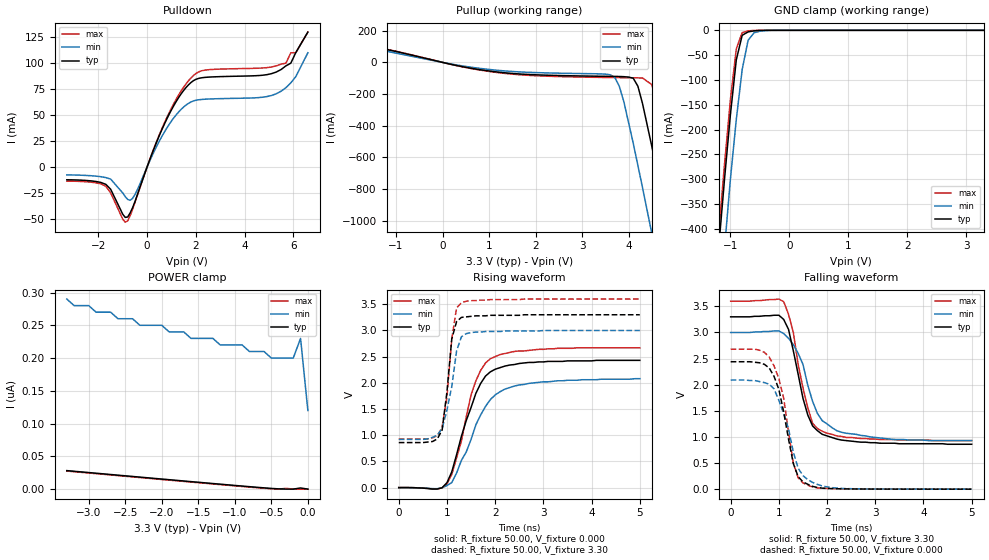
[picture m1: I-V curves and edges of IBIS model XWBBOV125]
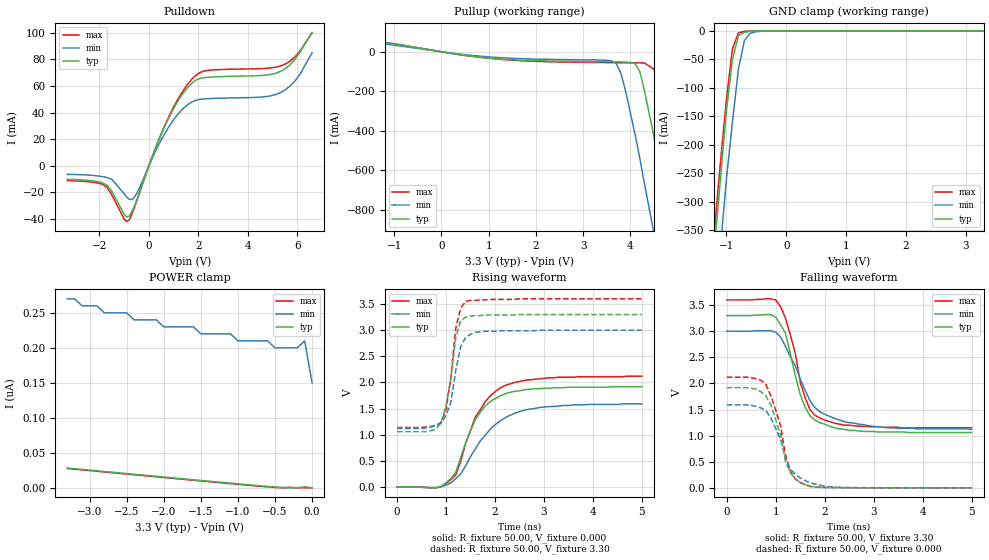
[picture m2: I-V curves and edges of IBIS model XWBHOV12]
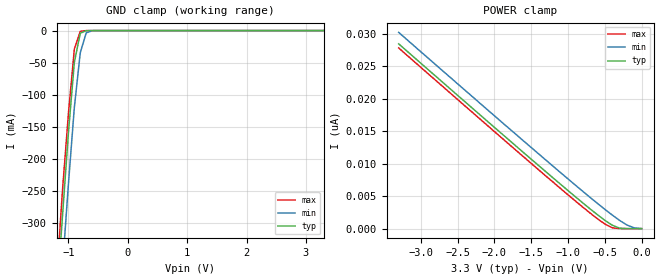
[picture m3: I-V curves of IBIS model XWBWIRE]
|   National Semiconductor Corporation
|   Networks Division
|   IBIS Model for DP83846A
|   80 Pin LQFP Package
| IBIS file dp83846a.ibs was created using s2ibis2 version 2.1
| North Carolina State University Electronics Research Laboratory 1997
| http://www.eigroup.org/ibis/tools.htm -> SPICE-toIBISconversion(IBISv2.1)
| s2ibis2.tar.Z   11FEB97   652K
| s2ibis2_fix.tar.Z 13MAY97   119K
[IBIS ver]   2.1
[File name]   dp83846a.ibs
[File Rev]   2.0
[Date]   17APR01
[Source]   National Semiconductor Corporation, Networks Division
[Notes]   For questions or comments contact
   Alan.E.Segervall@nsc.com or phone 408-721-7082
   Spectre s2ibis simulations, created by Alan E Segervall.
| Due to IBIS modeling limitations and design complexity this model
| does not support the Ethernet Transmit Data pins:
| [Pin]   signal_name   model_name
| 16  TD+   NC   0.321   4.888nH   0.078pF
| 17  TD-   NC   0.336   5.093nH   0.082pF
| Please refer to product datasheet and application notes for PC board
| layout recommendations.
[Disclaimer]  Absolutely no guarantees, for modeling purposes only.
   National Semiconductor Corporation hereby grants the user of this IBIS
model a non-exclusive, nontransferable license to use this IBIS model under
the following terms. Before using this IBIS model, the user should read this
license.  If the user does not accept these terms,  the IBIS model should be
returned to National within 30 days.
   The user is granted this license only to use the IBIS model and is not
granted rights to sell, load, rent, lease or license the IBIS model in whole
or in part, or in modified form to anyone other than user. User may modify
the IBIS model to suit its specific applications but rights to derivative
works and such modifications shall belong to National.
   This IBIS model is provided on an "AS IS" basis and National makes
absolutely no warranty with respect to the information contained herein.
NATIONAL DISCLAIMS AND CUSTOMER WAIVES ALL WARRANTIES, EXPRESS OR IMPLIED,
INCLUDING WARRANTIES OF MERCHANTABILITY OR FITNESS FOR A PARTICULAR PURPOSE.
The entire risk as to quality and performance is with the Customer.
ACCORDINGLY, IN NO EVENT SHALL THE COMPANY BE LIABLE FOR ANY DAMAGES, WHETHER
IN CONTRACT OR COURT, INCLUDING ANY LOST PROFITS OR OTHER INCIDENTAL,
CONSEQUENTIAL, EXEMPLARY, OR PUNITIVE DAMAGES ARISING OUT OF THE USE OR
APPLICATION OF THE IBIS model provided in this package. Further, National
reserves the right to make changes without notice to any product herein to
improve reliability, function, or design. National does not convey any license
under patent rights or any other intellectual property rights, including those
of third parties.
   National is not obligated to provide maintenance or support
for the licensed IBIS model.
[Copyright]   Copyright 2001, National Semiconductor Corporation, All rights
   reserved
|   Component DP83846A
[Component]   DP83846A
[Manufacturer]   National Semiconductor Corporation
[Package]
| variable   typ   min   max
R_pkg   0.333   0.287   0.382
L_pkg   5.049nH   4.529nH   5.845nH
C_pkg   0.106pF   0.078pF   0.283pF
[Pin] signal_name   model_name   R_pin   L_pin   C_pin
1   RESERVED   NC   0.382   5.845nH   0.283pF
2   ANA_GND1   GND   0.375   5.634nH   0.109pF
3   RBIAS   XWBWIRE   0.362   5.447nH   0.089pF
4   ANA_VDD1   POWER   0.350   5.273nH   0.082pF
5   RESERVED   NC   0.340   5.129nH   0.080pF
6   ANA_GND2   GND   0.332   4.986nH   0.078pF
7   ANA_VDD2   POWER   0.326   4.877nH   0.078pF
8   RESERVED   XWBWIRE   0.320   4.796nH   0.082pF
9   ANA_GND3   GND   0.314   4.751nH   0.091pF
10  RD-   RD   0.304   4.746nH   0.091pF
11  RD+   RD   0.287   4.529nH   0.090pF
12  ANA_VDD3   POWER   0.297   4.540nH   0.089pF
13  ANA_GND4   GND   0.303   4.576nH   0.080pF
14  ANA_VDD4   POWER   0.306   4.650nH   0.079pF
15  ANA_GND5   GND   0.313   4.753nH   0.078pF
16  TD+   NC   0.321   4.888nH   0.078pF
17  TD-   NC   0.336   5.093nH   0.082pF
18  ANA_GND6   GND   0.350   5.279nH   0.089pF
19  SUB_GND1   GND   0.363   5.480nH   0.106pF
20  RESERVED   NC   0.371   5.716nH   0.281pF
21  RESERVED   XWBBOV125   0.382   5.845nH   0.283pF
22  RESERVED   XWBBOV125   0.375   5.634nH   0.109pF
23  CORE_GND1   GND   0.362   5.447nH   0.089pF
24  CORE_VDD1   POWER   0.350   5.273nH   0.082pF
25  AN_0   XWBBOV125   0.340   5.129nH   0.080pF
26  AN_1   XWBBOV125   0.332   4.986nH   0.078pF
27  AN_EN   XWBBOV62   0.326   4.877nH   0.078pF
28  LED_SPEED   XWBBOV62   0.320   4.796nH   0.082pF
29  LED_RX/PADDR4   XWBBOV62   0.314   4.751nH   0.091pF
30  LED_TX/PADDR3   XWBBOV62   0.304   4.746nH   0.091pF
31  LED_GDLNK/PADDR2   XWBBOV125   0.287   4.529nH   0.090pF
32  LED_COL/PADDR1   XWBBOV62   0.297   4.540nH   0.089pF
33  LED_FDPLX/PADDR0   XWBBOV62   0.303   4.576nH   0.080pF
34  IO_GND   GND   0.306   4.650nH   0.079pF
35  IO_VDD   POWER   0.313   4.753nH   0.078pF
36  MDIO   XWBHOV12   0.321   4.888nH   0.078pF
37  MDC   XWBHOV12   0.336   5.093nH   0.082pF
38  RXD_3/CD_RF1   XWBBOV62   0.350   5.279nH   0.089pF
39  RXD_2/CD_RF0   XWBBOV62   0.363   5.480nH   0.106pF
40  RXD_1/CRM_LF_SEL   XWBBOV125   0.371   5.716nH   0.281pF
41  RXD_0/FCO_EN   XWBBOV125   0.382   5.845nH   0.283pF
42  IO_GND   GND   0.375   5.634nH   0.109pF
43  IO_VDD   POWER   0.362   5.447nH   0.089pF
44  RX_DV   XWBBOV62   0.350   5.273nH   0.082pF
45  RX_CLK   XWBBOV62   0.340   5.129nH   0.080pF
46  RX_ER/PAUSE_EN   XWBBOV62   0.332   4.986nH   0.078pF
47  RESERVED   XWBBOV125   0.326   4.877nH   0.078pF
48  CORE_GND2   GND   0.320   4.796nH   0.082pF
49  CORE_VDD2   POWER   0.314   4.751nH   0.091pF
50  TX_ER   XWBHOV12   0.304   4.746nH   0.091pF
51  TX_CLK   XWBHOV12   0.287   4.529nH   0.090pF
52  TX_EN   XWBHOV12   0.297   4.540nH   0.089pF
53  IO_GND3   GND   0.303   4.576nH   0.080pF
54  TXD_0   XWBHOV12   0.306   4.650nH   0.079pF
55  TXD_1   XWBHOV12   0.313   4.753nH   0.078pF
56  IO_GND4   GND   0.321   4.888nH   0.078pF
57  IO_VDD4   POWER   0.336   5.093nH   0.082pF
58  TXD_2   XWBHOV12   0.350   5.279nH   0.089pF
59  TXD_3   XWBHOV12   0.363   5.480nH   0.106pF
60  COL   XWBHOV12   0.371   5.716nH   0.281pF
61  CRS/LED_CFG   XWBHOV12   0.382   5.845nH   0.283pF
62  RESET   XWBHOV12   0.375   5.634nH   0.109pF
63  RESERVED   XWBHOV12   0.362   5.447nH   0.089pF
64  IO_GND5   GND   0.350   5.273nH   0.082pF
65  IO_VDD5   POWER   0.340   5.129nH   0.080pF
66  X2   OSC25_XO   0.332   4.986nH   0.078pF
67  X1   OSC25_XI   0.326   4.877nH   0.078pF
68  RESERVED   XWBHOV12   0.320   4.796nH   0.082pF
69  RESERVED   XWBHOV12   0.314   4.751nH   0.091pF
70  RESERVED   XWBHOV12   0.304   4.746nH   0.091pF
71  RESERVED   XWBHOV12   0.287   4.529nH   0.090pF
72  CORE_VDD3   POWER   0.297   4.540nH   0.089pF
73  CORE_GND3   GND   0.303   4.576nH   0.080pF
74  RESERVED   NC   0.306   4.650nH   0.079pF
75  RESERVED   NC   0.313   4.753nH   0.078pF
76  SUB_GND2   GND   0.321   4.888nH   0.078pF
77  RESERVED   NC   0.336   5.093nH   0.082pF
78  RESERVED   NC   0.350   5.279nH   0.089pF
79  SUB_GND3   GND   0.363   5.480nH   0.106pF
80  RESERVED   NC   0.371   5.716nH   0.281pF
[Diff Pin]  inv_pin  vdiff   tdelay_typ
11   10   0.100V   0.000s
16   17   0.000V   0.000s
| Models and submodels in the file (7): XWBBOV125 (I/O), XWBHOV12 (I/O), XWBWIRE (Input), RD (Input), XWBBOV62 (I/O), OSC25_XO (Output), OSC25_XI (Input)
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|   Model XWBBOV125
[Model]   XWBBOV125
Model_type   I/O
Polarity   Non-Inverting
Enable   Active-High
Vinl =   0.80V
Vinh =   2.00V
Vmeas =   1.50V
Cref =  20.00pF
Rref = 100.00k
C_comp   5.00pF   5.00pF   5.00pF
[Temperature Range]   25.00   0.14k   0.000
[Voltage Range]   3.30V   3.00V   3.60V
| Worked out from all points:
|   slope of the pulldown table from 0 to 0.495 V, typ, clamps not added: 16.5 ohm
|   slope of the pullup table from 0 to 0.495 V, typ, clamps not added: 16.1 ohm
|   GND clamp passes 1 mA (typ) near -0.58 V on its own axis
|   rising waveform, R_fixture 50.00, V_fixture 0.000: 20-80 % time 519ps typ, 631ps min, 459ps max; typ from 0 V to 2.43 V
|   rising waveform, R_fixture 50.00, V_fixture 3.30: 20-80 % time 163ps typ, 237ps min, 185ps max; typ from 0.86 V to 3.3 V
|   falling waveform, R_fixture 50.00, V_fixture 3.30: 20-80 % time 374ps typ, 469ps min, 351ps max; typ from 3.3 V to 0.86 V
|   falling waveform, R_fixture 50.00, V_fixture 0.000: 20-80 % time 318ps typ, 383ps min, 304ps max; typ from 2.44 V to 0 V
[Pulldown]
| voltage   I(typ)   I(min)   I(max)
-3.3V     -12.55mA   -7.84mA    -13.87mA
-1.7V     -16.93mA   -10.43mA   -18.73mA
-1V       -45.94mA   -25.36mA   -50.67mA
-800mV    -48.46mA   -31.53mA   -52.2mA
-500mV    -33.54mA   -26.73mA   -34.28mA
700mV     40.82mA    33.24mA    41.89mA
1.8V      81.34mA    62.58mA    85.74mA
5.3V      91.41mA    70.44mA    97.34mA
5.7V      97.44mA    76.39mA    100mA
5.9V      100mA      81mA       110mA
6.1V      110mA      86.86mA    110mA
6.6V      130mA      110mA      130mA
[Pullup]
| voltage   I(typ)   I(min)   I(max)
-3.3V     200mA      170mA      210mA
900mV     -50.23mA   -41.2mA    -52.73mA
3.6V      -88.17mA   -77.79mA   -95.51mA
3.8V      -89.02mA   -150mA     -96.22mA
3.9V      -90.24mA   -250mA     -96.54mA
4.1V      -99.71mA   -510mA     -97.17mA
4.3V      -260mA     -790mA     -98.85mA
4.5V      -530mA     -1.08A     -140mA
4.9V      -1.12A     -1.67A     -650mA
5.1V      -1.42A     -1.97A     -950mA
5.3V      -1.73A     -2.28A     -1.25A
6.6V      -3.73A     -4.26A     -3.25A
[GND_clamp]
| voltage   I(typ)   I(min)   I(max)
-3.3V     -3.64A     -3.72A     -3.62A
-1.2V     -440mA     -570mA     -410mA
-1.1V     -300mA     -440mA     -270mA
-1V       -170mA     -300mA     -140mA
-900mV    -59.59mA   -180mA     -37.47mA
-800mV    -10.05mA   -78.91mA   -4.5mA
-700mV    -3.19mA    -20.3mA    -1.15mA
-600mV    -1.14mA    -5.01mA    -210uA
-500mV    -210uA     -1.78mA    -18.22uA
-200mV    -44.3nA    -11.19uA   -980pA
3.3V      93.97pA    200nA      36.14pA
[POWER_clamp]
| voltage   I(typ)   I(min)   I(max)
-3.3V     28.33nA    290nA      27.68nA
-2.7V     22.38nA    270nA      21.73nA
-2.6V     21.39nA    260nA      20.74nA
-2.4V     19.41nA    260nA      18.76nA
-2.3V     18.42nA    250nA      17.77nA
-2V       15.46nA    250nA      14.81nA
-1.6V     11.54nA    230nA      10.88nA
-900mV    4.78nA     220nA      4.12nA
-500mV    1.18nA     200nA      630pA
-200mV    120pA      200nA      190pA
-100mV    1.86nA     230nA      45.35pA
0V        93.97pA    120nA      39.6pA
[Ramp]
| variable   typ   min   max
dV/dt_r   1.92/0.26n   1.74/0.34n   2.10/0.26n
dV/dt_f   1.92/0.27n   1.73/0.37n   2.10/0.26n
R_load = 0.50k
[Rising Waveform]
R_fixture = 50.00
V_fixture = 0.000
V_fixture_min = 0.000
V_fixture_max = 0.000
| time   V(typ)   V(min)   V(max)
0s        130uV      110uV      140uV
800ps     -25.56mV   -20.49mV   -29.57mV
1ns       93.95mV    39.4mV     72.64mV
1.1ns     300mV      96.74mV    250mV
1.3ns     980mV      520mV      890mV
1.5ns     1.53V      920mV      1.77V
1.6ns     1.8V       1.2V       2.04V
1.9ns     2.21V      1.68V      2.46V
2.7ns     2.39V      1.99V      2.62V
5ns       2.43V      2.08V      2.67V
[Rising Waveform]
R_fixture = 50.00
V_fixture = 3.30
V_fixture_min = 3.00
V_fixture_max = 3.60
| time   V(typ)   V(min)   V(max)
0s        860mV      920mV      930mV
700ps     880mV      960mV      950mV
800ps     930mV      1V         990mV
900ps     1.1V       1.13V      1.15V
1ns       1.83V      1.48V      1.74V
1.1ns     2.84V      1.93V      2.84V
1.2ns     3.17V      2.61V      3.43V
1.3ns     3.25V      2.88V      3.53V
1.8ns     3.28V      2.98V      3.58V
5ns       3.3V       3V         3.6V
[Falling Waveform]
R_fixture = 50.00
V_fixture = 3.30
V_fixture_min = 3.00
V_fixture_max = 3.60
| time   V(typ)   V(min)   V(max)
0s        3.3V       3V         3.6V
1.1ns     3.25V      2.98V      3.59V
1.2ns     3.06V      2.89V      3.35V
1.3ns     2.65V      2.77V      3V
1.5ns     1.74V      2.39V      1.94V
1.6ns     1.42V      1.99V      1.56V
1.7ns     1.21V      1.68V      1.26V
1.8ns     1.12V      1.45V      1.16V
2.4ns     930mV      1.07V      990mV
5ns       860mV      930mV      930mV
[Falling Waveform]
R_fixture = 50.00
V_fixture = 0.000
V_fixture_min = 0.000
V_fixture_max = 0.000
| time   V(typ)   V(min)   V(max)
0s        2.44V      2.09V      2.68V
600ps     2.42V      2.06V      2.66V
900ps     2.16V      1.92V      2.36V
1ns       1.91V      1.7V       2.12V
1.1ns     1.48V      1.45V      1.74V
1.3ns     490mV      710mV      500mV
1.4ns     240mV      400mV      220mV
1.5ns     140mV      260mV      120mV
2.2ns     8.79mV     21.51mV    9.2mV
5ns       240uV      370uV      270uV
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|   Model XWBHOV12
[Model]   XWBHOV12
Model_type   I/O
Polarity   Non-Inverting
Enable   Active-High
Vinl =   0.80V
Vinh =   2.00V
Vmeas =   1.50V
Cref =  20.00pF
Rref = 100.00k
C_comp   5.00pF   5.00pF   5.00pF
[Temperature Range]   25.00   0.14k   0.000
[Voltage Range]   3.30V   3.00V   3.60V
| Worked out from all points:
|   slope of the pulldown table from 0 to 0.495 V, typ, clamps not added: 21.1 ohm
|   slope of the pullup table from 0 to 0.495 V, typ, clamps not added: 28 ohm
|   GND clamp passes 1 mA (typ) near -0.60 V on its own axis
|   rising waveform, R_fixture 50.00, V_fixture 0.000: 20-80 % time 551ps typ, 775ps min, 585ps max; typ from 0 V to 1.92 V
|   rising waveform, R_fixture 50.00, V_fixture 3.30: 20-80 % time 212ps typ, 237ps min, 193ps max; typ from 1.06 V to 3.3 V
|   falling waveform, R_fixture 50.00, V_fixture 3.30: 20-80 % time 397ps typ, 612ps min, 395ps max; typ from 3.3 V to 1.06 V
|   falling waveform, R_fixture 50.00, V_fixture 0.000: 20-80 % time 336ps typ, 408ps min, 340ps max; typ from 1.92 V to 0 V
[Pulldown]
| voltage   I(typ)   I(min)   I(max)
-3.3V     -10.21mA   -6.41mA    -11.24mA
-1.7V     -14.38mA   -8.76mA    -15.95mA
-900mV    -38.4mA    -23.38mA   -41.84mA
-700mV    -34.77mA   -25.38mA   -36.84mA
-500mV    -26.29mA   -20.89mA   -26.78mA
800mV     35.83mA    29.09mA    36.68mA
1.3V      52.23mA    41.38mA    54.01mA
1.8V      62.95mA    48.5mA     66.19mA
2.4V      66.48mA    50.41mA    71.64mA
5.3V      70.67mA    54.75mA    74.83mA
5.9V      79.7mA     63.54mA    81.56mA
6.6V      100mA      84.8mA     100mA
[Pullup]
| voltage   I(typ)   I(min)   I(max)
-3.3V     110mA      27.65mA    110mA
-2.7V     96.2mA     77.73mA    99.58mA
1V        -31.19mA   -25.59mA   -32.8mA
3.6V      -50.7mA    -46.05mA   -54.92mA
3.8V      -51.25mA   -110mA     -55.32mA
4.1V      -59.9mA    -420mA     -55.87mA
4.3V      -200mA     -670mA     -57.12mA
4.5V      -430mA     -920mA     -88.04mA
4.9V      -950mA     -1.44A     -540mA
5.1V      -1.21A     -1.7A      -800mA
5.3V      -1.48A     -1.97A     -1.06A
6.6V      -3.23A     -3.7A      -2.81A
[GND_clamp]
| voltage   I(typ)   I(min)   I(max)
-3.3V     -3.18A     -3.26A     -3.16A
-1.2V     -380mA     -500mA     -350mA
-1.1V     -260mA     -380mA     -230mA
-1V       -140mA     -260mA     -120mA
-900mV    -50.62mA   -160mA     -31.57mA
-800mV    -8.35mA    -67.12mA   -3.69mA
-700mV    -2.68mA    -16.92mA   -950uA
-600mV    -980uA     -4.21mA    -170uA
-500mV    -190uA     -1.55mA    -15.48uA
-200mV    -43.2nA    -10.78uA   -890pA
3.3V      110pA      200nA      36.28pA
[POWER_clamp]
| voltage   I(typ)   I(min)   I(max)
-3.3V     28.34nA    270nA      27.68nA
-2.8V     23.38nA    250nA      22.72nA
-2V       15.48nA    230nA      14.81nA
-1.6V     11.55nA    230nA      10.88nA
-1.5V     10.58nA    220nA      9.91nA
-1.1V     6.7nA      220nA      6.03nA
-1V       5.74nA     210nA      5.07nA
-600mV    2.04nA     210nA      1.4nA
-500mV    1.2nA      200nA      630pA
-200mV    130pA      200nA      130pA
-100mV    1.59nA     210nA      43.62pA
0V        110pA      150nA      39.7pA
[Ramp]
| variable   typ   min   max
dV/dt_r   1.88/0.28n   1.69/0.38n   2.06/0.28n
dV/dt_f   1.90/0.29n   1.72/0.41n   2.08/0.28n
R_load = 0.50k
[Rising Waveform]
R_fixture = 50.00
V_fixture = 0.000
V_fixture_min = 0.000
V_fixture_max = 0.000
| time   V(typ)   V(min)   V(max)
0s        89.13uV    78.2uV     98.24uV
800ps     -12.15mV   -8.36mV    -14.42mV
1.1ns     160mV      77.86mV    140mV
1.2ns     280mV      160mV      230mV
1.4ns     840mV      400mV      830mV
1.6ns     1.29V      730mV      1.34V
1.9ns     1.63V      1.1V       1.74V
2.2ns     1.78V      1.32V      1.94V
3.1ns     1.89V      1.54V      2.09V
5ns       1.92V      1.59V      2.12V
[Rising Waveform]
R_fixture = 50.00
V_fixture = 3.30
V_fixture_min = 3.00
V_fixture_max = 3.60
| time   V(typ)   V(min)   V(max)
0s        1.06V      1.12V      1.14V
600ps     1.06V      1.13V      1.15V
900ps     1.23V      1.22V      1.24V
1ns       1.55V      1.37V      1.48V
1.1ns     2.08V      1.62V      2.09V
1.2ns     2.86V      2.23V      3.04V
1.3ns     3.18V      2.68V      3.42V
1.4ns     3.25V      2.86V      3.55V
1.8ns     3.29V      2.98V      3.58V
5ns       3.3V       3V         3.6V
[Falling Waveform]
R_fixture = 50.00
V_fixture = 3.30
V_fixture_min = 3.00
V_fixture_max = 3.60
| time   V(typ)   V(min)   V(max)
0s        3.3V       3V         3.6V
1ns       3.27V      2.98V      3.6V
1.2ns     2.96V      2.71V      3.25V
1.4ns     2.15V      2.34V      2.58V
1.5ns     1.79V      2.09V      2.03V
1.6ns     1.55V      1.87V      1.73V
1.7ns     1.38V      1.67V      1.5V
1.9ns     1.25V      1.46V      1.34V
2.9ns     1.08V      1.19V      1.17V
5ns       1.06V      1.12V      1.15V
[Falling Waveform]
R_fixture = 50.00
V_fixture = 0.000
V_fixture_min = 0.000
V_fixture_max = 0.000
| time   V(typ)   V(min)   V(max)
0s        1.92V      1.59V      2.12V
500ps     1.91V      1.58V      2.11V
800ps     1.76V      1.48V      1.98V
900ps     1.59V      1.34V      1.77V
1.1ns     1.01V      930mV      1.19V
1.2ns     500mV      560mV      630mV
1.3ns     290mV      360mV      320mV
1.5ns     110mV      190mV      100mV
2.2ns     5.47mV     13.63mV    5.12mV
5ns       120uV      180uV      150uV
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|   Model XWBWIRE
[Model]   XWBWIRE
Model_type   Input
Vinl =   0.80V
Vinh =   2.00V
Vmeas =   1.50V
Cref =  10.00pF
Rref =  50.00
C_comp   5.00pF   5.00pF   5.00pF
[Temperature Range]   27.00   100.00   0.000
[Voltage Range]   3.30V   3.00V   3.60V
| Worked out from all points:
|   GND clamp passes 1 mA (typ) near -0.72 V on its own axis
[GND_clamp]
| voltage   I(typ)   I(min)   I(max)
-3.3V     -3.63A     -3.7A      -3.6A
-1.2V     -420mA     -510mA     -390mA
-1.1V     -290mA     -370mA     -250mA
-1V       -160mA     -240mA     -130mA
-900mV    -49.63mA   -120mA     -28.72mA
-800mV    -4.09mA    -34.4mA    -1.19mA
-700mV    -130uA     -3.55mA    -25.7uA
-600mV    -3.97uA    -220uA     -540nA
3.3V      3.3pA      1.28nA     3pA
[POWER_clamp]
| voltage   I(typ)   I(min)   I(max)
-3.3V     28.41nA    30.17nA    27.78nA
-1.4V     9.72nA     11.51nA    9.06nA
-600mV    2.15nA     3.89nA     1.52nA
-500mV    1.29nA     2.98nA     720pA
-400mV    540pA      2.11nA     140pA
-300mV    83.01pA    1.28nA     9.12pA
-200mV    6.78pA     570pA      4.11pA
-100mV    3.6pA      120pA      3.85pA
0V        3.3pA      12.61pA    3.6pA
